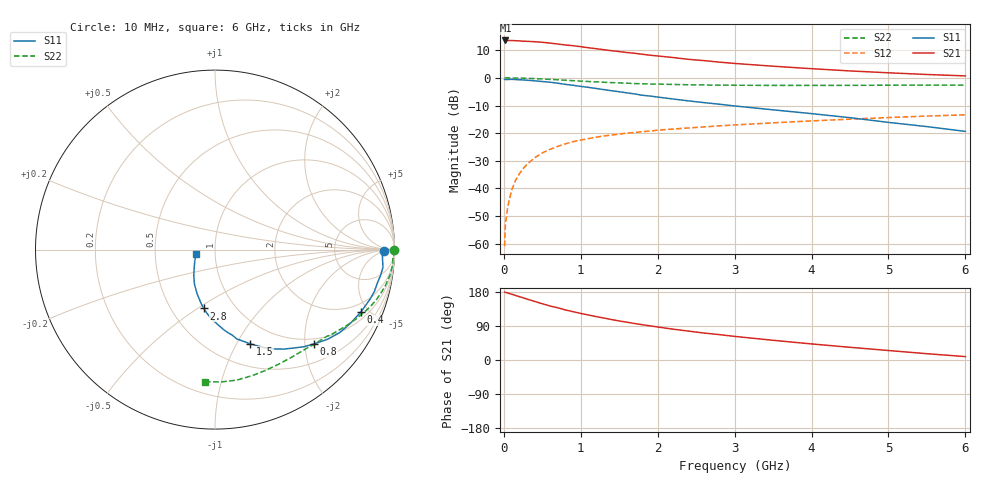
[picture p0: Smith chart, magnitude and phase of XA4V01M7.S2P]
! SIEMENS Discrete & RF Semiconductors
! BFY180
! Si NPN RF Bipolar Junction Transistor in MICRO-X
! VCE = 4 V  IC = 1.7 mA
! Common Emitter S-Parameters:  May  1997
# GHz  S  MA  R  50
!  f  S11  S21  S12  S22
! GHz  MAG  ANG  MAG  ANG  MAG  ANG  MAG  ANG
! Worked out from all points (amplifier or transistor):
!   36 points, 10 MHz to 6 GHz, reference 50 ohm
!   highest |S21| = 13.5 dB at 20 MHz (marker M1)
!   |S21| within 3 dB of that: start of sweep to 1.204 GHz
!   unconditionally stable (mu >= 1): 3.138 GHz to end of sweep
!   at 250 MHz: K = 0.11, MSG = 23.1 dB, |S12| = -32.9 dB
!   at 1.4 GHz: K = 0.62, MSG = 15.3 dB, |S12| = -20.7 dB
!   at 6 GHz: K = 1.06, MAG = 5.5 dB, |S12| = -13.4 dB
!   S11 on the Smith chart (normalised r, x): 10 MHz: 33, -5; 400 MHz: 1.40, -4.45; 800 MHz: 0.88, -2.21; 1.5 GHz: 0.74, -1.14; 2.8 GHz: 0.72, -0.53; 6 GHz: 0.81, -0.04
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0.01  0.9415 -0.5  4.721 179.1  0.0009 102.3  0.9959 -0.2
0.02  0.9327 -1.1  4.755 178.4  0.0022 95.1  0.9999 -0.6
0.05  0.9342 -2.9  4.724 176.9  0.0046 85.7  0.9967 -1.6
0.1  0.9411 -6.0  4.744 173.7  0.0092 87.0  0.9919 -3.1
0.15  0.933 -9.1  4.706 170.5  0.0138 84.7  0.9948 -4.7
0.25  0.9182 -14.7  4.602 164.2  0.0227 80.7  0.9875 -7.8
0.4  0.884 -23.2  4.509 154.6  0.0358 75.0  0.9695 -12.2
0.5  0.8584 -28.7  4.407 148.5  0.0438 71.0  0.9543 -14.9
0.6  0.8345 -33.7  4.259 142.5  0.0508 68.3  0.9399 -17.5
0.8  0.7628 -43.5  3.939 132.1  0.0638 62.9  0.9064 -22.2
0.9  0.7339 -47.5  3.822 127.5  0.0701 59.9  0.8894 -24.3
1.1  0.6733 -55.4  3.507 118.8  0.0796 55.9  0.8601 -28.1
1.2  0.643 -59.4  3.372 114.5  0.0845 54.0  0.8466 -30.0
1.5  0.5612 -69.5  2.991 103.0  0.0961 49.1  0.8101 -34.9
1.8  0.4842 -78.8  2.675 93.1  0.1062 46.0  0.7824 -39.1
2.2  0.4144 -88.4  2.334 81.4  0.1186 41.7  0.7605 -44.6
2.6  0.3569 -97.3  2.055 71.2  0.1296 38.7  0.7445 -49.7
2.8  0.3337 -100.8  1.928 67.0  0.1352 37.4  0.7391 -52.2
3.5  0.2641 -112.3  1.626 52.0  0.1535 32.4  0.7302 -60.8
4.5  0.1904 -128.4  1.336 33.5  0.1789 25.3  0.7322 -73.7
5.5  0.1312 -149.6  1.152 16.6  0.2035 17.7  0.7385 -87.6
6  0.1075 -167.0  1.085 9.0  0.2146 13.6  0.7376 -94.5
